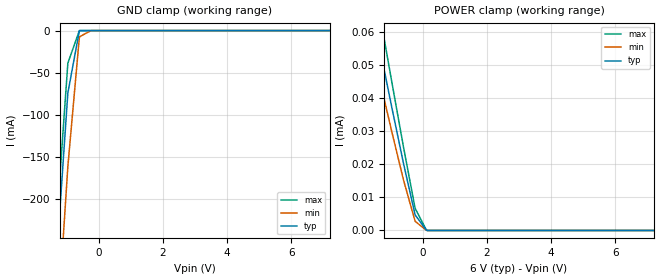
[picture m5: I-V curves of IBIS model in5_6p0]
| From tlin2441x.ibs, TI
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|   in5_6p0 Model
[Model]   in5_6p0
Model_type   Input
Vinl = 3
Vinh = 4
|   typ   min   max
C_comp   6.977pF   6.944pF   6.977pF
|  Where Nom  PVT is Nominal Process, 6.0V,   27C
|   Fast PVT is Strong Process,  6.5,   -40C
|   Slow PVT is Weak Process,   5.5V,   150C
[Model spec]
|subparameter
Vinl   3   2.5   3.5
Vinh   4   3.5   4.5
[Voltage Range]   6   5.5   6.5
|Junction Temperature
[Temperature Range]   27   150   -40
[Power Clamp Reference]   6   5.5   6.5
[GND Clamp Reference]   0   0   0
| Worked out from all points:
|   GND clamp passes 1 mA (typ) near -0.60 V on its own axis
[GND Clamp]
|   Voltage   I(typ)   I(min)   I(max)
-6V       -3.227A    -3.36A     -3.346A
-1.5V     -381.6mA   -483.7mA   -339.9mA
-1.32V    -274.7mA   -373mA     -233.6mA
-1.248V   -234.6mA   -330.6mA   -194.6mA
-996mV    -94.18mA   -182.5mA   -58.11mA
-960mV    -74.12mA   -161.4mA   -38.61mA
-600mV    -24.08uA   -7.461mA   -12.95uA
-240mV    -366.3nA   -1.564uA   -470.7nA
12V       0A         0A         0A
[POWER Clamp]
|   Voltage   I(typ)   I(min)   I(max)
-6V       281.9uA    247.4uA    326.2uA
-2.022V   87.77uA    74.08uA    103.1uA
-1.68V    71.23uA    59.56uA    84.05uA
-1.5V     62.58uA    51.98uA    74.09uA
-1.32V    53.92uA    44.41uA    64.13uA
-1.248V   50.5uA     41.43uA    60.19uA
-960mV    36.81uA    29.51uA    44.44uA
-600mV    20.11uA    15.13uA    25.04uA
-240mV    4.703uA    2.767uA    6.672uA
102mV     207.4nA    113.1nA    302.5nA
138mV     0A         0A         0A
12V       0A         0A         0A
